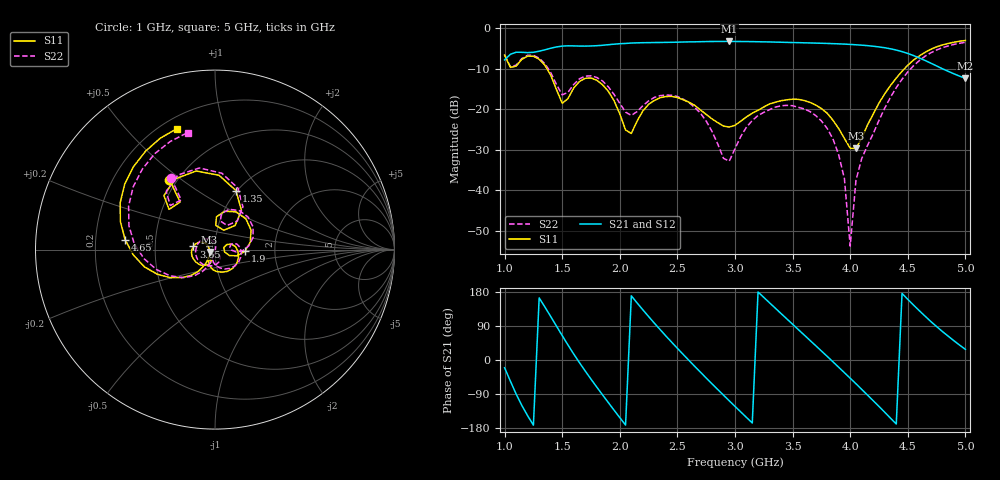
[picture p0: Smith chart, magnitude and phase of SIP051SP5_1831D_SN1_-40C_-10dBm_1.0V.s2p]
# GHz  S  dB  R  50
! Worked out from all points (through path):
!   81 points, 1 GHz to 5 GHz, reference 50 ohm
!   highest |S21| = -3.24 dB at 2.95 GHz (marker M1); lowest = -12.4 dB at 5 GHz (marker M2)
!   lowest |S11| = -29.7 dB at 4.05 GHz (marker M3), VSWR 1.07, Z = 47.1 - j1.22 ohm
!   |S11| at or under -10 dB: 1.368 GHz to 4.471 GHz (3.103 GHz wide, 106 % of centre)
!   |S22| runs from -53.8 to -3.5 dB; largest |S21 - S12| = 0.0019
!   S11 on the Smith chart (normalised r, x): 1 GHz: 0.45, +0.45; 1.35 GHz: 0.99, +0.74; 1.9 GHz: 1.40, -0.03; 3.65 GHz: 0.78, +0.03; 4.65 GHz: 0.33, +0.05; 5 GHz: 0.26, +0.70
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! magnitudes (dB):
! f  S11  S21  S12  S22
! 1 GHz  -6.6  -7.8  -7.8  -6.6
! 1.05 GHz  -9.7  -6.4  -6.4  -9.5
! 1.2 GHz  -6.9  -6.0  -6.0  -6.7
! 1.35 GHz  -9.1  -5.3  -5.3  -8.8
! 1.5 GHz  -18.5  -4.4  -4.4  -16.4
! 1.7 GHz  -12.4  -4.4  -4.4  -11.8
! 1.9 GHz  -15.6  -4.1  -4.1  -14.5
! 2.1 GHz  -26.0  -3.7  -3.7  -21.5
! 2.35 GHz  -17.2  -3.5  -3.5  -16.6
! 2.65 GHz  -19.0  -3.4  -3.3  -19.6
! 2.95 GHz  -24.4  -3.2  -3.2  -32.8
! 3 GHz  -24.0  -3.3  -3.3  -29.8
! 3.25 GHz  -19.4  -3.4  -3.4  -20.8
! 3.65 GHz  -18.3  -3.6  -3.6  -20.6
! 3.7 GHz  -19.0  -3.7  -3.7  -21.5
! 3.9 GHz  -24.8  -3.9  -3.9  -31.2
! 3.95 GHz  -27.2  -3.9  -3.9  -37.2
! 4 GHz  -29.6  -4.0  -4.0  -53.8
! 4.05 GHz  -29.7  -4.1  -4.1  -37.6
! 4.35 GHz  -14.1  -5.1  -5.1  -17.0
! 4.65 GHz  -6.0  -8.0  -8.0  -6.9
! 5 GHz  -3.0  -12.4  -12.4  -3.5
